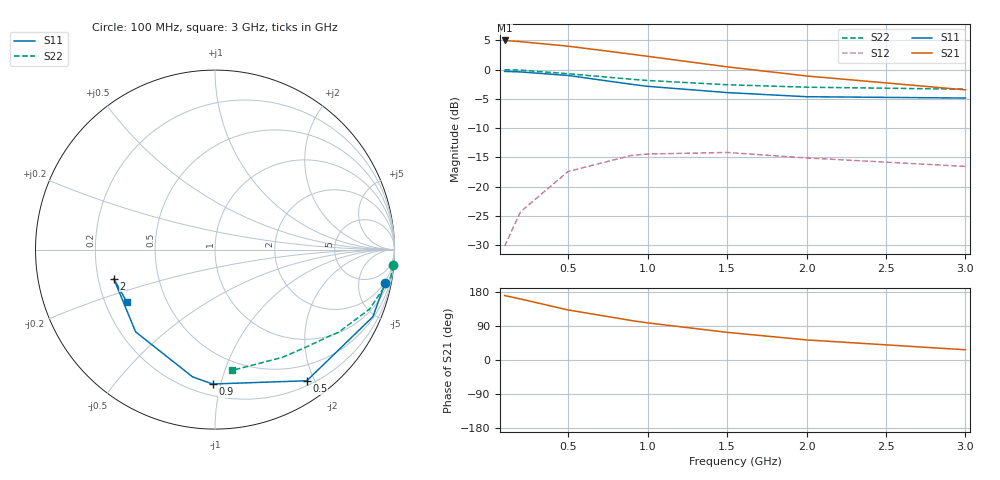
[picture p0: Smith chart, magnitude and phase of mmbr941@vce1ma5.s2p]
# MHz S MA R 50
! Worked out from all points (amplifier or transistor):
!   8 points, 100 MHz to 3 GHz, reference 50 ohm
!   highest |S21| = 5.0 dB at 100 MHz (marker M1)
!   |S21| within 3 dB of that: start of sweep to 1.081 GHz
!   unconditionally stable (mu >= 1): 1.99 GHz to end of sweep
!   at 200 MHz: K = 0.09, MSG = 14.5 dB, |S12| = -24.3 dB
!   at 1 GHz: K = 0.50, MSG = 8.4 dB, |S12| = -14.4 dB
!   at 3 GHz: K = 1.72, MAG = 1.6 dB, |S12| = -16.5 dB
!   S11 on the Smith chart (normalised r, x): 100 MHz: 2, -10; 500 MHz: 0.26, -1.89; 900 MHz: 0.28, -0.94; 2 GHz: 0.27, -0.13; 3 GHz: 0.29, -0.26
100  0.966 -11.0  1.776 170.0  0.031 83.0  0.998 -5.0
200  0.956 -23.0  1.735 161.0  0.061 75.0  0.991 -9.0
500  0.892 -55.0  1.587 132.0  0.135 55.0  0.923 -21.0
900  0.749 -91.0  1.355 104.0  0.185 35.0  0.827 -34.0
1000  0.72 -100.0  1.3 98.0  0.19 32.0  0.808 -36.0
1500  0.637 -134.0  1.057 73.0  0.196 18.0  0.743 -47.0
2000  0.587 -164.0  0.883 53.0  0.176 12.0  0.708 -58.0
3000  0.572 -149.0  0.672 27.0  0.149 33.0  0.68 -82.0
